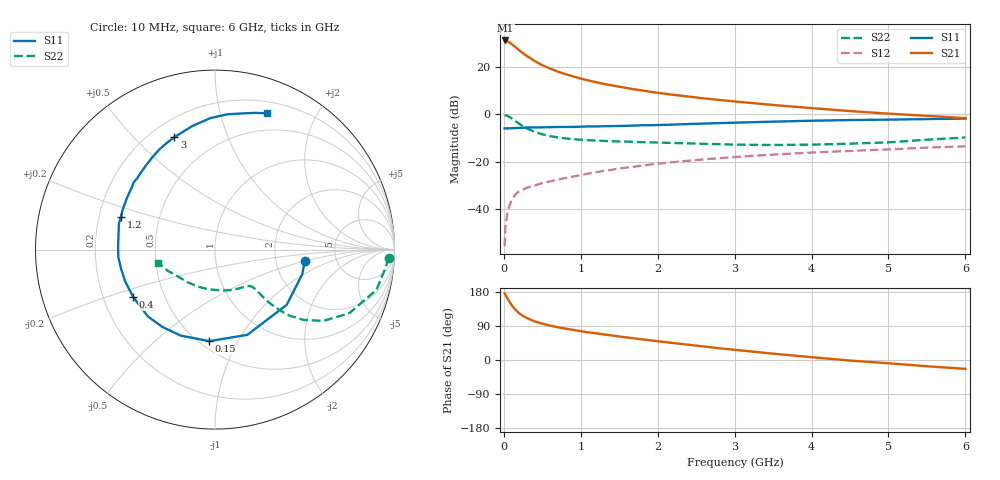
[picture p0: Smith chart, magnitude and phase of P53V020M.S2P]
! SIEMENS Small Signal Semiconductors
! BFP183
! Si NPN RF Bipolar Junction Transistor in SOT143
! VCE = 3 V  IC = 20 mA
! Common Emitter S-Parameters:  March  1996
# GHz  S  MA  R  50
!  f  S11  S21  S12  S22
! GHz  MAG  ANG  MAG  ANG  MAG  ANG  MAG  ANG
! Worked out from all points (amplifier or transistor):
!   36 points, 10 MHz to 6 GHz, reference 50 ohm
!   highest |S21| = 31.4 dB at 20 MHz (marker M1)
!   |S21| within 3 dB of that: start of sweep to 157.8 MHz
!   unconditionally stable (mu >= 1): 801.7 MHz to 5.557 GHz
!   at 250 MHz: K = 0.49, MSG = 28.9 dB, |S12| = -31.9 dB
!   at 1.4 GHz: K = 1.14, MAG = 15.7 dB, |S12| = -23.5 dB
!   at 6 GHz: K = 0.96, MSG = 6.0 dB, |S12| = -13.6 dB
!   S11 on the Smith chart (normalised r, x): 10 MHz: 2.93, -0.52; 150 MHz: 0.56, -0.77; 400 MHz: 0.33, -0.24; 1.2 GHz: 0.29, +0.15; 3 GHz: 0.29, +0.66; 6 GHz: 0.31, +1.41
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0.01  0.5042 -7.5  36.93 176.0  0.0016 89.3  0.9688 -2.7
0.02  0.5052 -15.8  36.95 172.4  0.004 89.1  0.9573 -5.7
0.05  0.5043 -37.6  35.51 161.1  0.009 79.3  0.9271 -14.0
0.1  0.508 -69.2  31.09 145.3  0.0152 64.3  0.8275 -25.4
0.15  0.5112 -93.6  26.8 132.7  0.0201 57.5  0.7218 -33.4
0.2  0.5158 -111.8  22.93 123.3  0.0234 53.1  0.6302 -38.4
0.25  0.5213 -124.4  19.69 116.1  0.0255 50.6  0.5589 -41.4
0.3  0.5276 -135.0  17.23 110.7  0.0279 49.0  0.5014 -43.0
0.4  0.5269 -150.0  13.55 102.0  0.0309 48.7  0.4243 -44.4
0.5  0.5307 -160.6  11.06 95.9  0.0351 48.8  0.3769 -44.6
0.6  0.5341 -168.4  9.401 90.8  0.0379 49.9  0.3452 -44.5
0.7  0.5403 -175.4  8.07 86.5  0.0411 51.4  0.3241 -44.4
0.9  0.5417 173.7  6.385 79.6  0.0481 52.1  0.2977 -44.8
1.1  0.555 164.7  5.243 73.0  0.0555 53.1  0.2827 -46.0
1.2  0.5543 160.9  4.802 70.4  0.0594 52.9  0.2781 -46.9
1.7  0.5788 143.2  3.391 56.9  0.078 52.0  0.2607 -53.9
2.2  0.6069 129.2  2.603 44.8  0.0968 48.7  0.2471 -63.5
3  0.666 109.9  1.879 26.9  0.1245 42.1  0.2279 -83.7
3.5  0.7005 100.3  1.58 16.7  0.1401 37.9  0.2241 -98.7
4.5  0.7569 84.8  1.174 -1.5  0.1676 28.9  0.2389 -131.0
5.5  0.7936 73.7  0.928 -16.5  0.1974 21.1  0.2899 -156.1
6  0.8136 69.0  0.831 -23.5  0.2097 16.5  0.3233 -167.0
